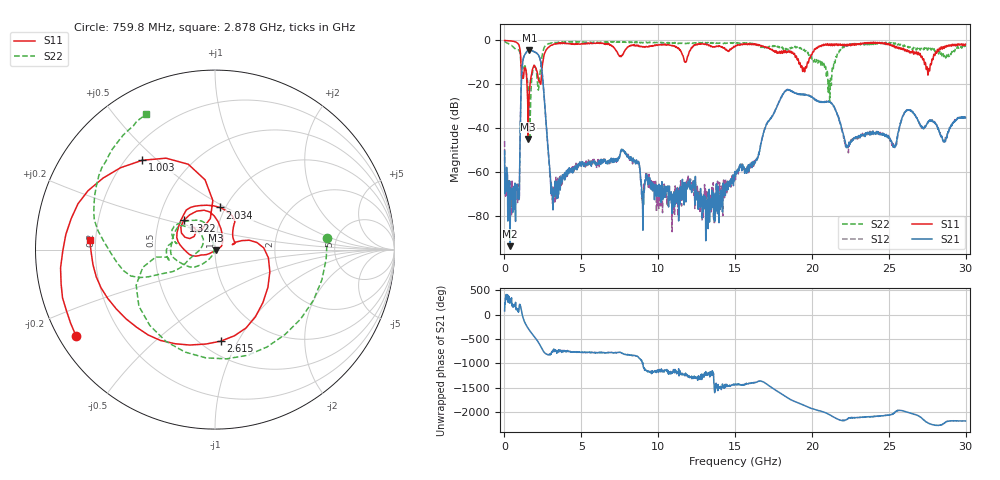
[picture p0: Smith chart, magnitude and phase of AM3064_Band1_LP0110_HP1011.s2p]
# Hz S DB R 50.0
!freq dBS11 angS11 dBS21 angS21 dBS12 angS12 dBS22 angS22
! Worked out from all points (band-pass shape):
!   1600 points, 10 MHz to 29.98 GHz, reference 50 ohm
!   highest |S21| = -4.50 dB at 1.622 GHz (marker M1); lowest = -93.9 dB at 366.1 MHz (marker M2)
!   |S21| within 3 dB of the highest: 1.258 GHz to 2.266 GHz (1.008 GHz wide, 57.2 % of centre)
!   lowest |S11| = -44.9 dB at 1.547 GHz (marker M3), VSWR 1.01, Z = 50.3 - j0.487 ohm
!   |S11| at or under -10 dB: 1.071 GHz to 2.494 GHz (1.423 GHz wide, 79.9 % of centre); 19.14 GHz to 19.7 GHz (561.8 MHz wide, 2.89 % of centre); 27.38 GHz to 27.78 GHz (407.1 MHz wide, 1.48 % of centre)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
!   |S22| runs from -46.0 to -0.4 dB; largest |S21 - S12| = 0.0082
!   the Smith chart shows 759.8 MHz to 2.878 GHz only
!   S11 on the Smith chart (normalised r, x): 759.8 MHz: 0.05, -0.28; 1.003 GHz: 0.27, +0.45; 1.322 GHz: 0.67, +0.23; 2.034 GHz: 0.94, +0.47; 2.615 GHz: 0.62, -0.85; 2.878 GHz: 0.18, +0.04
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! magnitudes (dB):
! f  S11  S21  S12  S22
! 10 MHz  0.0  -50.5  -45.9  -0.4
! 366.1 MHz  -0.2  -93.9  -70.3  -1.9
! 759.8 MHz  -0.8  -67.6  -72.5  -4.0
! 1.003 GHz  -3.9  -51.0  -51.3  -5.5
! 1.322 GHz  -12.4  -6.5  -6.4  -11.6
! 1.547 GHz  -44.9  -4.7  -4.6  -22.1
! 1.622 GHz  -23.1  -4.5  -4.5  -29.4
! 2.034 GHz  -12.5  -5.5  -5.5  -12.5
! 2.615 GHz  -5.8  -28.8  -28.7  -2.9
! 2.878 GHz  -3.1  -52.3  -53.6  -1.4
! 3.178 GHz  -1.8  -73.2  -68.3  -1.2
! 5.015 GHz  -1.6  -56.5  -56.6  -0.6
! 7.751 GHz  -5.8  -50.7  -50.4  -0.6
! 10 GHz  -2.1  -66.0  -73.6  -1.0
! 13.24 GHz  -2.0  -85.9  -68.5  -1.0
! 15 GHz  -2.8  -60.5  -61.4  -1.4
! 18.25 GHz  -4.9  -23.2  -23.2  -4.3
! 19.99 GHz  -6.5  -25.9  -25.9  -8.2
! 21.15 GHz  -1.8  -28.1  -28.1  -27.7
! 22.28 GHz  -2.5  -47.8  -48.3  -2.0
! 25 GHz  -1.5  -44.2  -44.7  -1.2
! 29.98 GHz  -1.7  -35.4  -35.3  -2.9
